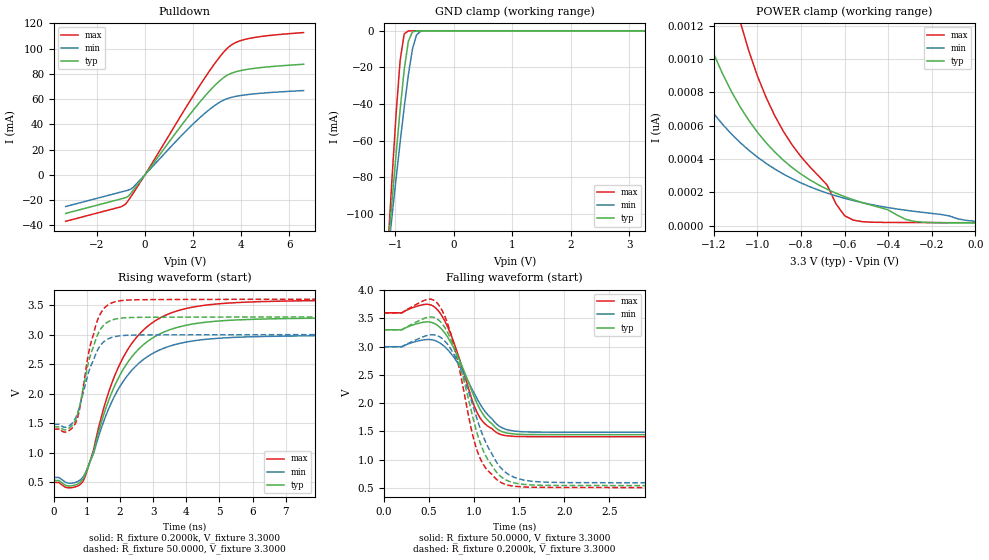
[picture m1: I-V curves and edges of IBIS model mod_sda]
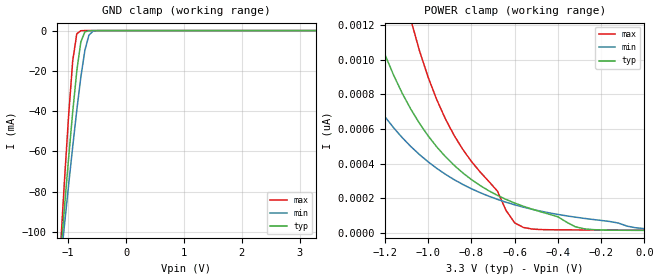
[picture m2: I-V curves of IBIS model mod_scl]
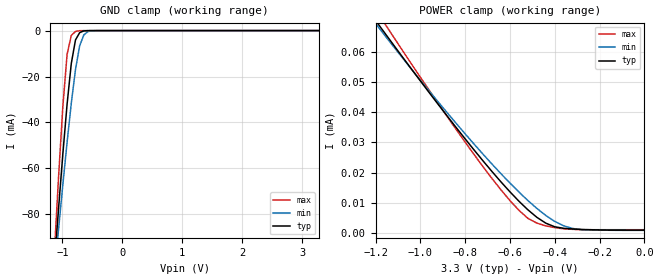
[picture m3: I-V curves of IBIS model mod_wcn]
| IBIS (I/O, Buffer, Information, Specification) Model, officially
| electronic behavioral standard for Buffer structures of digital pins.
[IBIS ver]  4.0
[File name] m24m04e_3d3_tssop8.ibs
[File Rev]  1.0
[Date]   13 Oct 2026
[Source]   CAD & Design Services (Catania) - STMicroelectronics
[Notes]
   (Note1)  This IBIS model includes the TSSOP8 package parasitic data
   (Note2)  This IBIS model has zero Notes and zero Warnings
[Disclaimer]
   Customers are solely responsible for all aspects of their
   own product designs or applications using this IBIS Model.
   STMicroelectronics assumes no liability for Custmer Designs
   and applications associated to this IBIS Model.
   In the use of this IBIS Model Customer shall not modify,
   disassemble, alter this Model in whole or in part.
   If Customers do not accept these terms, the IBIS Model
   may not be used. For any problems or modifications please
   contact STMicroelectronics (www.st.com).
[Copyright] (c) 2026 STMicroelectronics
|   Component M24M04E
[Component] M24M04E
[Manufacturer] STMicroelectronics
[Package]
| variable  typ   min   max
R_pkg   0.0   0.0   0.0
L_pkg   0.0H   0.0H   0.0H
C_pkg   0.0F   0.0F   0.0F
[Pin]  signal_name   model_name   R_pin   L_pin   C_pin
1   NC   NC   0.0   0.0   0.0
2   NC   NC   0.0   0.0   0.0
3   NC   NC   0.0   0.0   0.0
4   VSS   GND   0.0   0.0   0.0
5   SDA   mod_sda   0.0   0.0   0.0
6   SCL   mod_scl   0.0   0.0   0.0
7   WCN   mod_wcn   0.0   0.0   0.0
8   VCC   POWER   0.0   0.0   0.0
[Package Model]  182696_TSSOP8
[Define Package Model]  182696_TSSOP8
[Manufacturer]  STMicroelectronics
[OEM]  STMicroelectronics
[Description]  8 pin TSSOP package
[Number Of Pins]  8
[Pin Numbers]
|Pin Num   Terminal Name
1   | net1
2   | net2
3   | net3
4   | net4_GND
5   | net5
6   | net6
7   | net7
8   | net8_VDD
[Model Data]
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[End Model Data]
[End Package Model]
| Models and submodels in the file (3): mod_sda (I/O_open_drain), mod_scl (Input), mod_wcn (Input)
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|   Model mod_sda
[Model]   mod_sda
Model_type I/O_open_drain
Polarity   Inverting
Enable   Active-High
Vinl   =   0.990V
Vinh   =   2.310V
Vmeas  =   1.650V
Cref   =   30pF
Rref   =   500
Vref   =   3.300V
C_comp   4.846pF   4.640pF   4.858pF
[Temperature Range]  25.0000   85.0000   -40.0000
[Voltage Range]   3.3000V   3.0000V   3.6000V
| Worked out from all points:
|   slope of the pulldown table from 0 to 0.495 V, typ, clamps not added: 38.6 ohm
|   GND clamp passes 1 mA (typ) near -0.72 V on its own axis
|   rising waveform, R_fixture 0.2000k, V_fixture 3.3000: 20-80 % time 1.3ns typ, 1.31ns min, 1.29ns max; typ from 0.534 V to 3.28 V
|   rising waveform, R_fixture 50.0000, V_fixture 3.3000: 20-80 % time 483ps typ, 503ps min, 458ps max; typ from 1.44 V to 3.3 V
|   falling waveform, R_fixture 50.0000, V_fixture 3.3000: 20-80 % time 305ps typ, 333ps min, 275ps max; typ from 3.3 V to 1.44 V
|   falling waveform, R_fixture 0.2000k, V_fixture 3.3000: 20-80 % time 296ps typ, 338ps min, 259ps max; typ from 3.3 V to 0.535 V
[Pulldown]
|Voltage   I(typ)   I(min)   I(max)
-3.3V     -30.7mA    -25.23mA   -36.95mA
-1V       -19.2mA    -13.73mA   -25.45mA
-800mV    -18.11mA   -12.73mA   -23.16mA
-700mV    -17.15mA   -12.23mA   -20.6mA
-500mV    -12.56mA   -10.11mA   -14.89mA
1.4V      36.22mA    28.71mA    43.89mA
2.3V      58.05mA    45.54mA    71.37mA
3V        72.6mA     56.2mA     90.74mA
3.5V      79.7mA     60.87mA    101.6mA
3.9V      82.29mA    62.6mA     105.9mA
4.4V      84.03mA    63.87mA    108.4mA
6.6V      87.65mA    66.78mA    112.8mA
[GND_clamp]
|Voltage   I(typ)   I(min)   I(max)
-3.3V     -1.01A     -814.9mA   -1.404A
-1.13V    -120.1mA   -122.5mA   -118.8mA
-1.06V    -93.42mA   -101.5mA   -81.03mA
-990mV    -67.49mA   -80.83mA   -45.6mA
-920mV    -42.94mA   -60.76mA   -15.96mA
-850mV    -21.15mA   -41.63mA   -1.606mA
-780mV    -5.768mA   -24.18mA   -63.74uA
-710mV    -616.4uA   -10.08mA   -4.14uA
-640mV    -45.34uA   -2.266mA   -227.5nA
-570mV    -3.307uA   -288.2uA   -7.345nA
3.28V     15.71pA    85.37pA    15.34pA
[POWER_clamp]
|Voltage   I(typ)   I(min)   I(max)
-3.28V    8.108uA    4.441uA    13.9uA
-1.44V    2.157nA    1.226nA    5.11nA
-1.4V     1.906nA    1.108nA    4.359nA
-1.24V    1.164nA    741.3pA    2.31nA
-1.16V    911.1pA    607.7pA    1.684nA
-1.08V    714pA      499.1pA    1.229nA
-960mV    496.8pA    373.1pA    768.5pA
-880mV    391.1pA    308.5pA    563.5pA
-680mV    217.9pA    194.7pA    242.9pA
-600mV    173.5pA    163.3pA    59.05pA
-280mV    25.23pA    85.37pA    18.25pA
0V        15.81pA    26.21pA    16.88pA
[Ramp]
| variable   typ   min   max
dV/dt_r   1.1161/0.5213n   0.9100/0.5262n   1.3183/0.5287n
dV/dt_f   1.1164/0.3342n   0.9103/0.3515n   1.3185/0.3191n
R_load = 50.0000
[Rising Waveform]
R_fixture= 0.2000k
V_fixture= 3.3000
V_fixture_min= 3.0000
V_fixture_max= 3.6000
|time   V(typ)   V(min)   V(max)
0s        533.7mV    584.1mV    499.5mV
450ps     440mV      486.7mV    408.5mV
880ps     554.4mV    590.5mV    517.7mV
1.2ns     1.019V     984.4mV    1.05V
1.59ns    1.785V     1.656V     1.911V
1.96ns    2.276V     2.088V     2.461V
2.45ns    2.687V     2.453V     2.92V
3.15ns    2.996V     2.728V     3.262V
4.95ns    3.227V     2.936V     3.518V
10ns      3.284V     2.986V     3.583V
[Rising Waveform]
R_fixture= 50.0000
V_fixture= 3.3000
V_fixture_min= 3.0000
V_fixture_max= 3.6000
|time   V(typ)   V(min)   V(max)
0s        1.439V     1.483V     1.402V
400ps     1.397V     1.438V     1.359V
660ps     1.563V     1.592V     1.507V
800ps     1.841V     1.823V     1.804V
1.06ns    2.56V      2.38V      2.712V
1.27ns    2.924V     2.677V     3.16V
1.47ns    3.135V     2.857V     3.408V
1.75ns    3.244V     2.951V     3.535V
2.65ns    3.291V     2.993V     3.589V
10ns      3.298V     2.998V     3.598V
[Falling Waveform]
R_fixture= 50.0000
V_fixture= 3.3000
V_fixture_min= 3.0000
V_fixture_max= 3.6000
|time   V(typ)   V(min)   V(max)
0s        3.3V       3V         3.6V
200ps     3.3V       3V         3.6V
460ps     3.438V     3.126V     3.75V
580ps     3.394V     3.101V     3.678V
740ps     3.085V     2.889V     3.228V
980ps     2.199V     2.245V     2.05V
1.05ns    1.94V      2.032V     1.786V
1.23ns    1.58V      1.663V     1.503V
1.36ns    1.473V     1.534V     1.423V
10ns      1.44V      1.483V     1.403V
[Falling Waveform]
R_fixture= 0.2000k
V_fixture= 3.3000
V_fixture_min= 3.0000
V_fixture_max= 3.6000
|time   V(typ)   V(min)   V(max)
0s        3.3V       3V         3.6V
490ps     3.522V     3.204V     3.841V
610ps     3.469V     3.183V     3.738V
800ps     2.884V     2.79V      2.878V
970ps     1.858V     2.046V     1.539V
1.05ns    1.385V     1.638V     1.091V
1.23ns    819.7mV    1.008V     680.9mV
1.39ns    615.3mV    731.1mV    544.2mV
1.95ns    543.2mV    595.8mV    508.7mV
10ns      535.4mV    585.9mV    501.1mV
|   Model mod_scl
[Model]   mod_scl
Model_type Input
Vinl   =   0.990V
Vinh   =   2.310V
C_comp   3.680pF   3.516pF   3.856pF
[Temperature Range]  25.0000   85.0000   -40.0000
[Voltage Range]   3.3000V   3.0000V   3.6000V
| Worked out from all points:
|   GND clamp passes 1 mA (typ) near -0.72 V on its own axis
[GND_clamp]
|Voltage   I(typ)   I(min)   I(max)
-3.3V     -932.3mA   -765.4mA   -1.254A
-1.13V    -111.6mA   -115.5mA   -107.1mA
-1.06V    -86.89mA   -95.78mA   -73.35mA
-990mV    -62.95mA   -76.39mA   -41.66mA
-920mV    -40.25mA   -57.54mA   -14.95mA
-850mV    -20.05mA   -39.56mA   -1.583mA
-780mV    -5.606mA   -23.12mA   -63.7uA
-710mV    -613.7uA   -9.767mA   -4.14uA
-640mV    -45.33uA   -2.239mA   -227.5nA
-570mV    -3.307uA   -287.7uA   -7.345nA
3.28V     15.71pA    75.37pA    15.34pA
[POWER_clamp]
|Voltage   I(typ)   I(min)   I(max)
-3.28V    8.212uA    4.441uA    14.11uA
-1.44V    2.157nA    1.226nA    5.11nA
-1.4V     1.906nA    1.108nA    4.359nA
-1.24V    1.164nA    741.3pA    2.31nA
-1.16V    911.1pA    607.7pA    1.684nA
-1.08V    714pA      499.1pA    1.229nA
-960mV    496.8pA    373.1pA    768.5pA
-880mV    391.1pA    308.5pA    563.5pA
-680mV    217.9pA    194.7pA    242.9pA
-600mV    173.5pA    163.3pA    59.05pA
-280mV    25.23pA    85.37pA    18.25pA
0V        15.81pA    26.21pA    16.88pA
|   Model mod_wcn
[Model]   mod_wcn
Model_type Input
Vinl   =   0.990V
Vinh   =   2.310V
C_comp   3.680pF   3.516pF   3.856pF
[Temperature Range]  25.0000   85.0000   -40.0000
[Voltage Range]   3.3000V   3.0000V   3.6000V
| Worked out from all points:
|   GND clamp passes 1 mA (typ) near -0.71 V on its own axis
[GND_clamp]
|Voltage   I(typ)   I(min)   I(max)
-3.3V     -920.1mA   -753.8mA   -1.24A
-1.13V    -101.1mA   -105.4mA   -95.81mA
-1.06V    -76.85mA   -85.97mA   -62.9mA
-990mV    -53.6mA    -66.97mA   -32.91mA
-920mV    -32.13mA   -48.72mA   -10.45mA
-850mV    -14.39mA   -31.71mA   -2.152mA
-780mV    -4.089mA   -16.99mA   -383.7uA
-710mV    -886.5uA   -6.591mA   -37.2uA
-640mV    -124uA     -1.848mA   -14.71uA
-570mV    -19.8uA    -394.4uA   -11.19uA
-500mV    -9.874uA   -61.15uA   -9.456uA
3.28V     4.254uA    2.805uA    6.493uA
[POWER_clamp]
|Voltage   I(typ)   I(min)   I(max)
-3.28V    303.7uA    290.1uA    325.8uA
-1.2V     70.58uA    69.56uA    74.2uA
-1.16V    66.51uA    65.73uA    69.65uA
-1.12V    62.46uA    61.92uA    65.12uA
-880mV    38.76uA    39.86uA    38.58uA
-680mV    20.3uA     22.78uA    17.98uA
-600mV    13.56uA    16.48uA    10.65uA
-520mV    7.588uA    10.67uA    4.744uA
-440mV    3.142uA    5.7uA      2.232uA
-360mV    1.435uA    2.255uA    1.256uA
-320mV    1.205uA    1.377uA    1.093uA
0V        821nA      740nA      962.8nA
